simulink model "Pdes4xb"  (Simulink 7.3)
settings: Solver=ode45  StartTime=0.0  StopTime=50  RelTol=1e-3
undefined symbols (not defined in the file or in its folder): Aps, Bps, Cps, Dps, Kmix

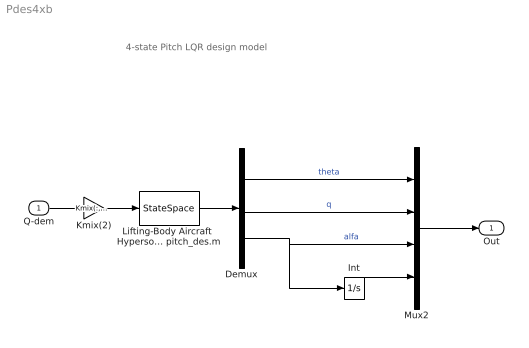
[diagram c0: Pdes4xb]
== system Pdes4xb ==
  note: 4-state Pitch LQR design model
  Q-dem : Inport  OutDataType=sfix(16)  OutScaling=2^0
  Demux : Demux  Outputs=3
  Int : Integrator
  Kmix(2) : Gain  Gain=Kmix(:,2)  ParameterDataType=sfix(16)  ParameterScaling=2^0  OutDataType=sfix(16)  OutScaling=2^0
  Lifting-Body Aircraft  Hypersonic Pitch  Design Model from file pitch_des.m : StateSpace  A=Aps  B=Bps  C=Cps  D=Dps
  Mux2 : Mux
  Out : Outport  OutDataType=sfix(16)  OutScaling=2^0
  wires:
  Lifting-Body Aircraft  Hypersonic Pitch  Design Model from file pitch_des.m/1 -> Demux/1
  Demux/2 -> Mux2/2  "q"
  Q-dem/1 -> Kmix(2)/1
  Demux/3 -> Mux2/3, Int/1  "alfa"
  Demux/1 -> Mux2/1  "theta"
  Kmix(2)/1 -> Lifting-Body Aircraft  Hypersonic Pitch  Design Model from file pitch_des.m/1
  Int/1 -> Mux2/4
  Mux2/1 -> Out/1
